| IBIS file stm32mp251_253_255_257_vfbga424.ibs
[IBIS ver] 5.1
[File name] stm32mp251_253_255_257_vfbga424.ibs
[File Rev] 1.3
[Date] 09-10-2025
[Source] Data Created at STMicroelectronics
[Notes]  File originated from ELDO simulations.
[Disclaimer]  This information is for modeling purpose only and is
   not guaranted. The information is subject to change without
   notice.
[Copyright] Copyright 2025 STMicroelectronics Inc.
|   Component stm32mp251_253_255_257_vfbga424
[Component] stm32mp25_505_tfbga14x14_424
[Manufacturer] stm32mp251_253_255_257_vfbga424
[Package]
| variable   typ   min   max
R_pkg   0.0   0.0   0.0
L_pkg   0.0H   0.0H   0.0H
C_pkg   0.0F   0.0F   0.0F
[Pin]  signal_name   model_name   R_pin   L_pin   C_pin
1A1  VSS  gnd
1A3  VSS  gnd
1A5  VSS  gnd
1A7  VSS  gnd
1A9  VSS  gnd
1A11  VSS  gnd
1B2  VSS  gnd
1B4  VSS  gnd
1B6  VSS  gnd
1B8  VSS  gnd
1B10  VSS  gnd
1B12  VSS  gnd
1C1  VDDCORE  nc
1C3  VDDCORE  nc
1C5  VDDCORE  nc
1C7  VDDCPU  nc
1C9  VDDCPU  nc
1C11  VDDQDDR  power
1D2  VDDCORE  nc
1D4  VDDCORE  nc
1D6  VDDCPU  nc
1D8  VDDCPU  nc
1D10  VDDCPU  nc
1D12  VDDQDDR  power
1E1  VDDA18PLL3  nc
1E3  VDDCORE  nc
1E5  VDDCORE  nc
1E7  VSS  gnd
1E9  VSS  gnd
1E11  VDDQDDR  power
1F2  VDDCORE  nc
1F4  VDDCORE  nc
1F6  VSS  gnd
1F8  VSS  gnd
1F10  VSS  gnd
1F12  VDDQDDR  power
1G1  VSS  gnd
1G3  VSS  gnd
1G5  VSS  gnd
1G7  VDDGPU  nc
1G9  VDDGPU  nc
1G11  VSS  gnd
1H2  VSS  gnd
1H4  VSS  gnd
1H6  VDDGPU  nc
1H8  VDDGPU  nc
1H10  VDDGPU  nc
1H12  VSS  gnd
1J1  VSS  gnd
1J3  VSS  gnd
1J5  VSS  gnd
1J7  VSS  gnd
1J9  VSS  gnd
1J11  VSS  gnd
1K2  VSS  gnd
1K4  VSS  gnd
1K6  VSS  gnd
1K8  VSS  gnd
1K10  VSS  gnd
1K12  VSS  gnd
1L1  VDD  power
1L3  VDD  power
1L5  VDD  power
1L7  VDDGPU  nc
1L9  VDDGPU  nc
1L11  VDDQDDR  power
1M2  VDD  power
1M4  VDD  power
1M6  VDDGPU  nc
1M8  VDDGPU  nc
1M10  VDDGPU  nc
1M12  VDDQDDR  power
A1  VSS  gnd
A2  VSS  gnd
A3  CSI_D0N  DPHY_IBIS_L1
A6  DSI_D3P  DPHY_IBIS
A7  DSI_D2N  DPHY_IBIS
A10  DSI_D1N  DPHY_IBIS
A11  PB11  io8_tt
A14  PB2  io8_tt
A15  PD11  io8_tt_i3c
A18  PD6  io8_tt
A19  PD1  io8_tt
A22  PE6  io8_tt
A23  PE9  io8_tt
A26  PB13  io8_tt
A27  VSS  gnd
AA1  OSC32_OUT  isudq_tt
AA2  OSC32_IN  isudq_tt
AA3  BOOT1  isudq_tt
AA5  JTCK_SWCLK  io8_tt
AA7  PG3  io8_tt
AA9  PC3  io8_tt
AA11  PF5  io8_tt
AA13  PH9  io8_tt
AA15  PF0  io8_tt_i3c
AA17  PA8  io8_tt_i3c
AA19  UCPD1_CC2  nc
AA21  DDR_A30  mal4drv20_PAD
AA23  DDR_A27  mal4drv20_PAD
AA25  DDR_DQS0P  mal4drv27_PAD
AA26  DDR_DQS0N  mal4drv27_PAD
AB1  BOOT2  isudq_tt
AB2  BOOT3  isudq_tt
AB3  VDDA18AON  power
AB4  PWR_CPUON  io8_tt
AB6  VDDA18ADC  power
AB8  PF7  io8_tt
AB10  PC6  io8_tt_i3c
AB12  PA14  io8_tt
AB14  PC0  io8_tt
AB16  PH4  io8_tt
AB18  UCPD1_CC1  nc
AB20  VDDCOMBOPHY  nc
AB22  VDDCOMBOPHYTX  nc
AB24  DDR_A26  mal4drv20_PAD
AB25  DDR_DQM0  mal4drv27_PAD
AB26  DDR_DQ0  mal4drv27_PAD
AB27  DDR_DQ2  mal4drv27_PAD
AC2  JTDO_TRACESWO  io8_tt
AC3  VSSAON  gnd
AC5  VSSA  nc
AC7  PF6  io8_tt
AC9  PC4  io8_tt
AC11  VSS  gnd
AC13  PA12  io8_tt_i3c
AC15  PF2  io8_tt_i3c
AC17  PH2  io8_tt_i3c
AC19  PA1  io8_tt_i3c
AC21  VDDPCIECLK  nc
AC23  DDR_A28  mal4drv20_PAD
AC25  DDR_A7  mal4drv20_PAD
AC26  DDR_DQ1  mal4drv27_PAD
AC27  DDR_DQ3  mal4drv27_PAD
AD3  PWR_ON  io8_tt
AD4  PG1  io8_tt_i3c
AD6  PG4  io8_tt
AD8  PC11  io8_tt
AD10  PC5  io8_tt_i3c
AD12  PA11  io8_tt
AD14  PA13  io8_tt
AD16  PH8  io8_tt
AD18  PA3  io8_tt_i3c
AD20  USB3DR_VBUS  nc
AD22  VDDA18USB  power
AD24  COMBOPHY_TX1N  synopsys_usb3_tx
AD25  DDR_A1  mal4drv20_PAD
AE1  NRST  nc
AE2  JTMS_SWDIO  io8_tt
AE3  JTDI  io8_tt
AE4  PF11  io8_tt
AE5  PF10  io8_tt
AE6  PB15  io8_tt
AE7  PC12  io8_tt_i3c
AE8  PF9  io8_tt
AE9  PC9  io8_tt
AE10  PF8  io8_tt
AE11  PF1  io8_tt
AE12  PC2  io8_tt
AE13  PA15  io8_tt_i3c
AE14  PH11  io8_tt
AE15  PA10  io8_tt
AE16  PH7  io8_tt_i3c
AE17  PA5  io8_tt
AE18  PA7  io8_tt
AE19  PH3  io8_tt_i3c
AE20  USBH_HS_TXRTUNE  nc
AE21  VDD33USB  power
AE22  VDD33UCPD  nc
AE23  VDDA18COMBOPHY  power
AE24  COMBOPHY_TX1P  synopsys_usb3_tx
AE25  PCIE_CLKINP  nc
AE26  PCIE_CLKINN  nc
AF1  PWR_LP  io8_tt
AF2  OSC_OUT  isudq_tt
AF3  NJTRST  io8_tt
AF5  PA0  io8_tt
AF6  VREFN  nc
AF7  PG0  io8_tt_i3c
AF9  PC7  io8_tt
AF10  PF4  io8_tt
AF11  PF3  io8_tt
AF13  PH12  io8_tt
AF14  PH10  io8_tt
AF15  PA9  io8_tt
AF17  PA2  io8_tt_i3c
AF18  PA6  io8_tt
AF19  PH6  io8_tt_i3c
AF21  USBH_HS_DP  USB2_HS_IBIS
AF22  USB3DR_DP  USB2_HS_IBIS
AF23  USB3DR_TXRTUNE  nc
AF25  COMBOPHY_RX1N  synopsys_usb3_rx
AF26  PCIE_CLKOUTP  nc
AF27  COMBOPHY_REXT  nc
AG1  VSS  gnd
AG2  OSC_IN  isudq_tt
AG5  PG2  io8_tt_i3c
AG6  VREFP  nc
AG9  PC8  io8_tt
AG10  PC10  io8_tt
AG13  PH13  io8_tt
AG14  PC1  io8_tt_i3c
AG17  PA4  io8_tt
AG18  PH5  io8_tt
AG21  USBH_HS_DM  USB2_HS_IBIS
AG22  USB3DR_DM  USB2_HS_IBIS
AG25  COMBOPHY_RX1P  synopsys_usb3_rx
AG26  PCIE_CLKOUTN  nc
AG27  VSS  gnd
B1  LVDS2_D0P  nc
B2  LVDS2_D0N  nc
B3  CSI_D0P  DPHY_IBIS_L1
B5  CSI_D1P  DPHY_IBIS_L1
B6  DSI_D3N  DPHY_IBIS
B7  DSI_D2P  DPHY_IBIS
B9  DSI_D0P  DPHY_IBIS
B10  DSI_D1P  DPHY_IBIS
B11  PB10  io8_tt
B13  PB0  io8_tt
B14  PB3  io8_tt
B15  PB4  io8_tt_i3c
B17  PD0  io8_tt
B18  PD5  io8_tt
B19  PE0  io8_tt
B21  PE4  io8_tt
B22  PE7  io8_tt
B23  PE11  io8_tt
B25  PE14  io8_tt
B26  PD12  io8_tt
B27  PI11  io8_tt
C2  LVDS2_D1P  nc
C3  LVDS2_D1N  nc
C4  CSI_CKP  DPHY_IBIS_L1
C5  CSI_D1N  DPHY_IBIS_L1
C6  VSS  gnd
C7  DSI_CKP  DPHY_IBIS
C8  DSI_CKN  DPHY_IBIS
C9  DSI_D0N  DPHY_IBIS
C10  VSS  gnd
C11  PB7  io8_tt
C12  PB1  io8_tt
C13  PB6  io8_tt
C14  PB5  io8_tt_i3c
C15  PD9  io8_tt
C16  PD8  io8_tt
C17  PD10  io8_tt_i3c
C18  PD4  io8_tt
C19  PE1  io8_tt
C20  PE2  io8_tt
C21  PE3  io8_tt
C22  PE5  io8_tt
C23  PE8  io8_tt
C24  PE13  io8_tt
C25  PE12  io8_tt
C26  PB12  io8_tt
C27  PB14  io8_tt
D3  LVDS2_D2N  nc
D4  CSI_CKN  DPHY_IBIS_L1
D6  DSI_REXT  nc
D8  PB8  io8_tt
D10  VDDIO3  power
D12  PD2  io8_tt
D14  VDDIO1  power
D16  PI10  io8_tt
D18  VDDIO2  power
D20  PD7  io8_tt
D22  PE10  io8_tt
D24  PE15  io8_tt
D25  PD13  io8_tt
E1  LVDS2_D3P  nc
E2  LVDS2_D3N  nc
E3  LVDS2_D2P  nc
E5  VDDCSI  nc
E7  VSS  gnd
E9  VDDIO4  power
E11  VDDIO3  power
E13  VDDIO1  power
E15  PD15  io8_tt_i3c
E17  VDDIO2  power
E19  PD14  io8_tt_i3c
E21  DDR_RESETN  nc
E23  DDR_A23  mal4drv20_PAD
E25  DDR_DQ19  mal4drv27_PAD
E26  DDR_DQ17  mal4drv27_PAD
F1  LVDS2_D4P  nc
F2  LVDS2_D4N  nc
F3  VSS  gnd
F4  VDDLVDS  nc
F6  CSI_REXT  nc
F8  VDDDSI  nc
F10  PB9  io8_tt
F12  VSS  gnd
F14  VSS  gnd
F16  VSS  gnd
F18  VDDCPU  nc
F20  VDDA18DDR  nc
F22  DDR_A22  mal4drv20_PAD
F24  DDR_DQ18  mal4drv27_PAD
F25  DDR_DQ16  mal4drv27_PAD
F26  DDR_DQS2N  mal4drv27_PAD
F27  DDR_DQS2P  mal4drv27_PAD
G2  LVDS1_D0P  nc
G3  LVDS1_D0N  nc
G5  VDDA18LVDS  power
G7  VDDA18CSI  power
G9  VDDA18DSI  power
G11  VDDIO4  power
G13  PD3  io8_tt
G15  VDDCPU  nc
G17  VDDCPU  nc
G19  VDDA18PLL1  nc
G21  DDR_VREF  nc
G23  DDR_A18  mal4drv20_PAD
G25  DDR_DQ23  mal4drv27_PAD
G26  DDR_DQ22  mal4drv27_PAD
G27  DDR_DQM2  mal4drv27_PAD
H3  LVDS1_D1P  nc
H4  LVDS1_D1N  nc
H6  VDDA18PLL2  nc
H22  DDR_A21  mal4drv20_PAD
H24  DDR_A17  mal4drv20_PAD
H25  DDR_DQ21  mal4drv27_PAD
J1  LVDS1_D2P  nc
J2  LVDS1_D2N  nc
J3  PI6  io8_tt
J5  PI7  io8_tt
J7  VSS  gnd
J21  DDR_A20  mal4drv20_PAD
J23  DDR_A16  mal4drv20_PAD
J25  DDR_DQ20  mal4drv27_PAD
J26  DDR_DQ24  mal4drv27_PAD
K1  LVDS1_D4P  nc
K2  LVDS1_D4N  nc
K3  VSS  gnd
K4  PI5  io8_tt
K6  PG15  io8_tt
K22  DDR_ZQ  nc
K24  DDR_A13  mal4drv20_PAD
K25  DDR_DQ25  mal4drv27_PAD
K26  DDR_DQ26  mal4drv27_PAD
K27  DDR_DQ27  mal4drv27_PAD
L2  LVDS1_D3P  nc
L3  LVDS1_D3N  nc
L5  PG8  io8_tt
L7  PI0  io8_tt
L21  DDR_A19  mal4drv20_PAD
L23  DDR_A12  mal4drv20_PAD
L25  DDR_DQ28  mal4drv27_PAD
L26  DDR_DQS3P  mal4drv27_PAD
L27  DDR_DQS3N  mal4drv27_PAD
M3  PG9  io8_tt
M4  PG10  io8_tt
M6  PI1  io8_tt_i3c
M22  VDDQDDR  power
M24  DDR_A14  mal4drv20_PAD
M25  DDR_DQM3  mal4drv27_PAD
N1  PG14  io8_tt
N2  PG11  io8_tt
N3  PG12  io8_tt
N5  PI2  io8_tt
N7  PI3  io8_tt
N21  VDDQDDR  power
N23  DDR_A15  mal4drv20_PAD
N25  DDR_DQ29  mal4drv27_PAD
N26  DDR_DQ30  mal4drv27_PAD
P1  PG13  io8_tt_i3c
P2  PF13  io8_tt
P3  PF14  io8_tt
P4  PF12  io8_tt
P6  PI4  io8_tt
P22  DDR_A3  mal4drv20_PAD
P24  DDR_A11  mal4drv20_PAD
P25  DDR_DQ31  mal4drv27_PAD
P26  DDR_DQ11  mal4drv27_PAD
P27  DDR_DQ10  mal4drv27_PAD
R2  PF15  io8_tt
R3  PG5  io8_tt_i3c
R5  PZ5  io8_tt
R7  V08CAP  nc
R21  VDDQDDR  power
R23  DDR_A10  mal4drv20_PAD
R25  DDR_DQS1N  mal4drv27_PAD
R26  DDR_DQ9  mal4drv27_PAD
R27  DDR_DQ8  mal4drv27_PAD
T3  PG6  io8_tt_i3c
T4  PZ0  io8_tt_i3c
T6  VBAT  power
T22  DDR_A9  mal4drv20_PAD
T24  DDR_A5  mal4drv20_PAD
T25  DDR_DQS1P  mal4drv27_PAD
U1  PI9  io8_tt
U2  PG7  io8_tt
U3  PZ9  io8_tt_i3c
U5  PI8  io8_tt
U7  PZ1  io8_tt_i3c
U21  DDR_A0  mal4drv20_PAD
U23  DDR_A4  mal4drv20_PAD
U25  DDR_DQ15  mal4drv27_PAD
U26  DDR_DQM1  mal4drv27_PAD
V1  PZ8  io8_tt
V2  PZ7  io8_tt
V3  PZ4  io8_tt_i3c
V4  PZ6  io8_tt
V6  VSS  gnd
V22  DDR_A8  mal4drv20_PAD
V24  DDR_A2  mal4drv20_PAD
V25  DDR_DQ14  mal4drv27_PAD
V26  DDR_DQ12  mal4drv27_PAD
V27  DDR_DQ13  mal4drv27_PAD
W2  PDR_ON  nc
W3  NRSTC1MS  io8_tt
W5  PZ2  io8_tt_i3c
W7  PC13  io8_tt
W21  DDR_A25  mal4drv20_PAD
W23  DDR_A31  mal4drv20_PAD
W25  DDR_DQ4  mal4drv27_PAD
W26  DDR_DQ6  mal4drv27_PAD
W27  DDR_DQ5  mal4drv27_PAD
Y3  BOOT0  isudq_tt
Y4  VSS  gnd
Y6  PZ3  io8_tt_i3c
Y22  DDR_A29  mal4drv20_PAD
Y24  DDR_A6  mal4drv20_PAD
Y25  DDR_DQ7  mal4drv27_PAD
[Package Model]   505-fcbga-14x14-424-240118v2
[Pin Mapping]   pulldown_ref   pullup_ref   | Comment
1A1  gnd  nc
1A3  gnd  nc
1A5  gnd  nc
1A7  gnd  nc
1A9  gnd  nc
1A11  gnd  nc
1B2  gnd  nc
1B4  gnd  nc
1B6  gnd  nc
1B8  gnd  nc
1B10  gnd  nc
1B12  gnd  nc
1C1  nc  nc
1C3  nc  nc
1C5  nc  nc
1C7  nc  nc
1C9  nc  nc
1C11  nc  vddqddr
1D2  nc  nc
1D4  nc  nc
1D6  nc  nc
1D8  nc  nc
1D10  nc  nc
1D12  nc  vddqddr
1E1  nc  nc
1E3  nc  nc
1E5  nc  nc
1E7  gnd  nc
1E9  gnd  nc
1E11  nc  vddqddr
1F2  nc  nc
1F4  nc  nc
1F6  gnd  nc
1F8  gnd  nc
1F10  gnd  nc
1F12  nc  vddqddr
1G1  gnd  nc
1G3  gnd  nc
1G5  gnd  nc
1G7  nc  nc
1G9  nc  nc
1G11  gnd  nc
1H2  gnd  nc
1H4  gnd  nc
1H6  nc  nc
1H8  nc  nc
1H10  nc  nc
1H12  gnd  nc
1J1  gnd  nc
1J3  gnd  nc
1J5  gnd  nc
1J7  gnd  nc
1J9  gnd  nc
1J11  gnd  nc
1K2  gnd  nc
1K4  gnd  nc
1K6  gnd  nc
1K8  gnd  nc
1K10  gnd  nc
1K12  gnd  nc
1L1  nc  vdd
1L3  nc  vdd
1L5  nc  vdd
1L7  nc  nc
1L9  nc  nc
1L11  nc  vddqddr
1M2  nc  vdd
1M4  nc  vdd
1M6  nc  nc
1M8  nc  nc
1M10  nc  nc
1M12  nc  vddqddr
A1  gnd  nc
A2  gnd  nc
A3  gnd  VDDA18CSI
A6  gnd  VDDA18DSI
A7  gnd  VDDA18DSI
A10  gnd  VDDA18DSI
A11  gnd  vddio4
A14  gnd  vddio4
A15  gnd  vddio3
A18  gnd  vddio3
A19  gnd  vddio3
A22  gnd  vddio2
A23  gnd  vddio2
A26  gnd  vdd
A27  gnd  nc
AA1  gnd  vdd  | Depending on IO usage
| AA1  gnd  vsw  | Depending on IO usage
AA2  gnd  vdd  | Depending on IO usage
| AA2  gnd  vsw  | Depending on IO usage
AA3  gnd  vdd
AA5  gnd  vdd
AA7  gnd  vdd  | Depending on IO usage
| AA7  gnd  vsw  | Depending on IO usage
AA9  gnd  vdd  | Depending on IO usage
| AA9  gnd  vsw  | Depending on IO usage
AA11  gnd  vdd
AA13  gnd  vdd
AA15  gnd  vdd
AA17  gnd  vdd
AA19  nc  nc
AA21  gnd  vddqddr
AA23  gnd  vddqddr
AA25  gnd  vddqddr
AA26  gnd  vddqddr
AB1  gnd  vdd
AB2  gnd  vdd
AB3  nc  vdda18aon
AB4  gnd  vdd
AB6  nc  vdda18adc
AB8  gnd  vdd  | Depending on IO usage
| AB8  gnd  vsw  | Depending on IO usage
AB10  gnd  vdd
AB12  gnd  vdd
AB14  gnd  vdd
AB16  gnd  vdd
AB18  nc  nc
AB20  nc  nc
AB22  nc  nc
AB24  gnd  vddqddr
AB25  gnd  vddqddr
AB26  gnd  vddqddr
AB27  gnd  vddqddr
AC2  gnd  vdd
AC3  gnd_aon  nc
AC5  nc  nc
AC7  gnd  vdd  | Depending on IO usage
| AC7  gnd  vsw  | Depending on IO usage
AC9  gnd  vdd  | Depending on IO usage
| AC9  gnd  vsw  | Depending on IO usage
AC11  gnd  nc
AC13  gnd  vdd
AC15  gnd  vdd
AC17  gnd  vdd
AC19  gnd  vdd
AC21  nc  nc
AC23  gnd  vddqddr
AC25  gnd  vddqddr
AC26  gnd  vddqddr
AC27  gnd  vddqddr
AD3  gnd  vdd
AD4  gnd  vdd  | Depending on IO usage
| AD4  gnd  vsw  | Depending on IO usage
AD6  gnd  vdd
AD8  gnd  vdd
AD10  gnd  vdd  | Depending on IO usage
| AD10  gnd  vsw  | Depending on IO usage
AD12  gnd  vdd
AD14  gnd  vdd
AD16  gnd  vdd
AD18  gnd  vdd
AD20  nc  nc
AD22  nc  vdda18usb
AD24  gnd  vdda18combophy
AD25  gnd  vddqddr
AE1  nc  nc
AE2  gnd  vdd
AE3  gnd  vdd
AE4  gnd  vdd
AE5  gnd  vdd
AE6  gnd  vdd
AE7  gnd  vdd
AE8  gnd  vdd
AE9  gnd  vdd
AE10  gnd  vdd
AE11  gnd  vdd
AE12  gnd  vdd
AE13  gnd  vdd
AE14  gnd  vdd
AE15  gnd  vdd
AE16  gnd  vdd
AE17  gnd  vdd
AE18  gnd  vdd
AE19  gnd  vdd
AE20  nc  nc
AE21  nc  VDD33USB
AE22  nc  nc
AE23  nc  vdda18combophy
AE24  gnd  vdda18combophy
AE25  nc  nc
AE26  nc  nc
AF1  gnd  vdd
AF2  gnd_aon  vdda18aon
AF3  gnd  vdd
AF5  gnd  vdd
AF6  nc  nc
AF7  gnd  vdd
AF9  gnd  vdd
AF10  gnd  vdd
AF11  gnd  vdd
AF13  gnd  vdd
AF14  gnd  vdd
AF15  gnd  vdd
AF17  gnd  vdd
AF18  gnd  vdd
AF19  gnd  vdd
AF21  gnd  VDD33USB
AF22  gnd  VDD33USB
AF23  nc  nc
AF25  gnd  vdda18combophy
AF26  nc  nc
AF27  nc  nc
AG1  gnd  nc
AG2  gnd_aon  vdda18aon
AG5  gnd  vdd
AG6  nc  nc
AG9  gnd  vdd
AG10  gnd  vdd
AG13  gnd  vdd
AG14  gnd  vdd
AG17  gnd  vdd
AG18  gnd  vdd
AG21  gnd  VDD33USB
AG22  gnd  VDD33USB
AG25  gnd  vdda18combophy
AG26  nc  nc
AG27  gnd  nc
B1  nc  nc
B2  nc  nc
B3  gnd  VDDA18CSI
B5  gnd  VDDA18CSI
B6  gnd  VDDA18DSI
B7  gnd  VDDA18DSI
B9  gnd  VDDA18DSI
B10  gnd  VDDA18DSI
B11  gnd  vddio4
B13  gnd  vddio4
B14  gnd  vddio4
B15  gnd  vddio4
B17  gnd  vddio3
B18  gnd  vddio3
B19  gnd  vddio1
B21  gnd  vddio1
B22  gnd  vddio2
B23  gnd  vddio2
B25  gnd  vddio2
B26  gnd  vdd
B27  gnd  vdd
C2  nc  nc
C3  nc  nc
C4  gnd  VDDA18CSI
C5  gnd  VDDA18CSI
C6  gnd  nc
C7  gnd  VDDA18DSI
C8  gnd  VDDA18DSI
C9  gnd  VDDA18DSI
C10  gnd  nc
C11  gnd  vddio4
C12  gnd  vddio4
C13  gnd  vddio4
C14  gnd  vddio4
C15  gnd  vddio3
C16  gnd  vddio3
C17  gnd  vddio3
C18  gnd  vddio3
C19  gnd  vddio1
C20  gnd  vddio1
C21  gnd  vddio1
C22  gnd  vddio1
C23  gnd  vddio2
C24  gnd  vddio2
C25  gnd  vddio2
C26  gnd  vdd
C27  gnd  vdd
D3  nc  nc
D4  gnd  VDDA18CSI
D6  nc  nc
D8  gnd  vddio4
D10  nc  vddio3
D12  gnd  vddio3
D14  nc  vddio1
D16  gnd  vdd
D18  nc  vddio2
D20  gnd  vddio3
D22  gnd  vddio2
D24  gnd  vddio2
D25  gnd  vdd
E1  nc  nc
E2  nc  nc
E3  nc  nc
E5  nc  nc
E7  gnd  nc
E9  nc  vddio4
E11  nc  vddio3
E13  nc  vddio1
E15  gnd  vdd
E17  nc  vddio2
E19  gnd  vdd
E21  nc  nc
E23  gnd  vddqddr
E25  gnd  vddqddr
E26  gnd  vddqddr
F1  nc  nc
F2  nc  nc
F3  gnd  nc
F4  nc  nc
F6  nc  nc
F8  nc  nc
F10  gnd  vddio4
F12  gnd  nc
F14  gnd  nc
F16  gnd  nc
F18  nc  nc
F20  nc  nc
F22  gnd  vddqddr
F24  gnd  vddqddr
F25  gnd  vddqddr
F26  gnd  vddqddr
F27  gnd  vddqddr
G2  nc  nc
G3  nc  nc
G5  nc  vdda18lvds
G7  nc  VDDA18CSI
G9  nc  VDDA18DSI
G11  nc  vddio4
G13  gnd  vddio3
G15  nc  nc
G17  nc  nc
G19  nc  nc
G21  nc  nc
G23  gnd  vddqddr
G25  gnd  vddqddr
G26  gnd  vddqddr
G27  gnd  vddqddr
H3  nc  nc
H4  nc  nc
H6  nc  nc
H22  gnd  vddqddr
H24  gnd  vddqddr
H25  gnd  vddqddr
J1  nc  nc
J2  nc  nc
J3  gnd  vdd
J5  gnd  vdd
J7  gnd  nc
J21  gnd  vddqddr
J23  gnd  vddqddr
J25  gnd  vddqddr
J26  gnd  vddqddr
K1  nc  nc
K2  nc  nc
K3  gnd  nc
K4  gnd  vdd
K6  gnd  vdd
K22  nc  nc
K24  gnd  vddqddr
K25  gnd  vddqddr
K26  gnd  vddqddr
K27  gnd  vddqddr
L2  nc  nc
L3  nc  nc
L5  gnd  vdd
L7  gnd  vdd
L21  gnd  vddqddr
L23  gnd  vddqddr
L25  gnd  vddqddr
L26  gnd  vddqddr
L27  gnd  vddqddr
M3  gnd  vdd
M4  gnd  vdd
M6  gnd  vdd
M22  nc  vddqddr
M24  gnd  vddqddr
M25  gnd  vddqddr
N1  gnd  vdd
N2  gnd  vdd
N3  gnd  vdd
N5  gnd  vdd
N7  gnd  vdd
N21  nc  vddqddr
N23  gnd  vddqddr
N25  gnd  vddqddr
N26  gnd  vddqddr
P1  gnd  vdd
P2  gnd  vdd
P3  gnd  vdd
P4  gnd  vdd
P6  gnd  vdd
P22  gnd  vddqddr
P24  gnd  vddqddr
P25  gnd  vddqddr
P26  gnd  vddqddr
P27  gnd  vddqddr
R2  gnd  vdd
R3  gnd  vdd
R5  gnd  vdd  | Depending on IO usage
| R5  gnd  vsw  | Depending on IO usage
R7  nc  nc
R21  nc  vddqddr
R23  gnd  vddqddr
R25  gnd  vddqddr
R26  gnd  vddqddr
R27  gnd  vddqddr
T3  gnd  vdd
T4  gnd  vdd  | Depending on IO usage
| T4  gnd  vsw  | Depending on IO usage
T6  nc  vsw
T22  gnd  vddqddr
T24  gnd  vddqddr
T25  gnd  vddqddr
U1  gnd  vdd
U2  gnd  vdd
U3  gnd  vdd
U5  gnd  vdd  | Depending on IO usage
| U5  gnd  vsw  | Depending on IO usage
U7  gnd  vdd  | Depending on IO usage
| U7  gnd  vsw  | Depending on IO usage
U21  gnd  vddqddr
U23  gnd  vddqddr
U25  gnd  vddqddr
U26  gnd  vddqddr
V1  gnd  vdd
V2  gnd  vdd
V3  gnd  vdd  | Depending on IO usage
| V3  gnd  vsw  | Depending on IO usage
V4  gnd  vdd  | Depending on IO usage
| V4  gnd  vsw  | Depending on IO usage
V6  gnd  nc
V22  gnd  vddqddr
V24  gnd  vddqddr
V25  gnd  vddqddr
V26  gnd  vddqddr
V27  gnd  vddqddr
W2  nc  nc
W3  gnd  vdd
W5  gnd  vdd  | Depending on IO usage
| W5  gnd  vsw  | Depending on IO usage
W7  gnd  vdd  | Depending on IO usage
| W7  gnd  vsw  | Depending on IO usage
W21  gnd  vddqddr
W23  gnd  vddqddr
W25  gnd  vddqddr
W26  gnd  vddqddr
W27  gnd  vddqddr
Y3  gnd  vdd
Y4  gnd  nc
Y6  gnd  vdd  | Depending on IO usage
| Y6  gnd  vsw  | Depending on IO usage
Y22  gnd  vddqddr
Y24  gnd  vddqddr
Y25  gnd  vddqddr
[Diff Pin]   inv_pin   vdiff   tdelay_typ   tdelay_min   tdelay_max
U23   T24   0.320V   0ns   NA   NA   |CKA
|J23   H24   0.320V   0ns   NA   NA   |CKB only in LPDDR4 32 bit
AA25   AA26   0.320V   0ns   NA   NA   |DQS0
T25   R25   0.320V   0ns   NA   NA   |DQS1
F27   F26   0.320V   0ns   NA   NA   |DQS2
L26   L27   0.320V   0ns   NA   NA   |DQS3
AG25   AF25   NA   NA   NA   NA
AE24   AD24   NA   NA   NA   NA
C4   D4   NA   NA   NA   NA
B3   A3   NA   NA   NA   NA
B5   C5   NA   NA   NA   NA
C7   C8   NA   NA   NA   NA  |DSI CKP CKN
B9   C9   400.000mV   0ns   NA   NA   |D0P D0N
B10   A10   400.000mV   0ns   NA   NA   |D1P D1N
B7   A7   400.000mV   0ns   NA   NA   |D2P D2N
A6   B6   400.000mV   0ns   NA   NA   |D3P D3N
G2   G3   NA   NA   NA   NA
H3   H4   NA   NA   NA   NA
J1   J2   NA   NA   NA   NA
L2   L3   NA   NA   NA   NA
K1   K2   NA   NA   NA   NA
B1   B2   NA   NA   NA   NA
C2   C3   NA   NA   NA   NA
E3   D3   NA   NA   NA   NA
E1   E2   NA   NA   NA   NA
F1   F2   NA   NA   NA   NA
AE25   AE26   NA   NA   NA   NA
AF26   AG26   NA   NA   NA   NA
AF22   AG22   NA   NA   NA   NA   |USB3DR_DP _DM
AF21   AG21   NA   NA   NA   NA   |USBH_HS_DP _DM
[Model Selector] DPHY_IBIS_L1
DPHY_RX_2P5G_L1   DPHY HSRX model at 2.5Gbps for lane 1
DPHY_RX_1P5G_L1   DPHY HSRX model at 1.5Gbps for lane 1
[Model Selector] DPHY_IBIS
DPHY_TX_2P5G   DPHY HSTX model at 2.5Gbps
DPHY_TX_1P5G   DPHY HSTX model at 1.5Gbps
[Model Selector] USB2_HS_IBIS
USB2_HSRX   USB2 HSRX model
USB2_HSTX_00_0_01_0011_11   TuningBits_AMP_PULSE_RISE_REF_XV=00_0_01_0011_11
USB2_HSTX_00_0_10_0101_11   TuningBits_AMP_PULSE_RISE_REF_XV=00_0_10_0101_11
USB2_HSTX_00_0_11_0111_11   TuningBits_AMP_PULSE_RISE_REF_XV=00_0_11_0111_11
USB2_HSTX_00_1_01_0011_11   TuningBits_AMP_PULSE_RISE_REF_XV=00_1_01_0011_11
USB2_HSTX_00_1_10_0101_11   TuningBits_AMP_PULSE_RISE_REF_XV=00_1_10_0101_11
USB2_HSTX_00_1_11_0111_11   TuningBits_AMP_PULSE_RISE_REF_XV=00_1_11_0111_11
USB2_HSTX_01_0_01_0011_11   TuningBits_AMP_PULSE_RISE_REF_XV=01_0_01_0011_11
USB2_HSTX_01_0_10_0101_11   TuningBits_AMP_PULSE_RISE_REF_XV=01_0_10_0101_11
USB2_HSTX_01_0_11_0111_11   TuningBits_AMP_PULSE_RISE_REF_XV=01_0_11_0111_11
USB2_HSTX_01_1_01_0011_11   TuningBits_AMP_PULSE_RISE_REF_XV=01_1_01_0011_11
USB2_HSTX_01_1_10_0101_11   TuningBits_AMP_PULSE_RISE_REF_XV=01_1_10_0101_11
USB2_HSTX_01_1_11_0111_11   TuningBits_AMP_PULSE_RISE_REF_XV=01_1_11_0111_11
USB2_HSTX_10_0_01_0011_11   TuningBits_AMP_PULSE_RISE_REF_XV=10_0_01_0011_11
USB2_HSTX_10_0_10_0101_11   TuningBits_AMP_PULSE_RISE_REF_XV=10_0_10_0101_11
USB2_HSTX_10_0_11_0111_11   TuningBits_AMP_PULSE_RISE_REF_XV=10_0_11_0111_11
USB2_HSTX_10_1_01_0011_11   TuningBits_AMP_PULSE_RISE_REF_XV=10_1_01_0011_11
USB2_HSTX_10_1_10_0101_11   TuningBits_AMP_PULSE_RISE_REF_XV=10_1_10_0101_11
USB2_HSTX_10_1_11_0111_11   TuningBits_AMP_PULSE_RISE_REF_XV=10_1_11_0111_11
[Model Selector] io8_tt
io8_tt_ls_3v3   "GPIO - 3V tolerant - 3.3V range - Low speed"
io8_tt_ms_3v3   "GPIO - 3V tolerant - 3.3V range - Med speed"
io8_tt_fs_3v3   "GPIO - 3V tolerant - 3.3V range - Fast speed"
io8_tt_hs_3v3   "GPIO - 3V tolerant - 3.3V range - High speed"
io8_tt_hslv_ls_1v8   "GPIO HSLV - 3V tolerant - 1.8V range - Low speed"
io8_tt_hslv_ms_1v8   "GPIO HSLV - 3V tolerant - 1.8V range - Med speed"
io8_tt_hslv_fs_1v8   "GPIO HSLV - 3V tolerant - 1.8V range - Fast speed"
io8_tt_hslv_hs_1v8   "GPIO HSLV - 3V tolerant - 1.8V range - High speed"
[Model Selector] io8_tt_i3c
io8_tt_ls_3v3   "GPIO - 3V tolerant - 3.3V range - Low speed"
io8_tt_ms_3v3   "GPIO - 3V tolerant - 3.3V range - Med speed"
io8_tt_fs_3v3   "GPIO - 3V tolerant - 3.3V range - Fast speed"
io8_tt_hs_3v3   "GPIO - 3V tolerant - 3.3V range - High speed"
io8_tt_hslv_ls_1v8   "GPIO HSLV - 3V tolerant - 1.8V range - Low speed"
io8_tt_hslv_ms_1v8   "GPIO HSLV - 3V tolerant - 1.8V range - Med speed"
io8_tt_hslv_fs_1v8   "GPIO HSLV - 3V tolerant - 1.8V range - Fast speed"
io8_tt_hslv_hs_1v8   "GPIO HSLV - 3V tolerant - 1.8V range - High speed"
io8_tt_i3c_3v3   "GPIO - 3V tolerant - 3.3V range - Open drain"
[Model Selector] isudq_tt
isudq_tt_1v8   "Input Buffer - 3V tolerant - 1.8V range"
isudq_tt_3v3   "Input Buffer - 3V tolerant - 3.3V range"
[Model Selector]   mal4drv20_PAD
mal4drv20_d3l_40   DDR3L mal4drv20 cell  Z0=40-Ohm Driver
mal4drv20_d3l_60   DDR3L mal4drv20 cell  Z0=60-Ohm Driver
mal4drv20_d3l_120   DDR3L mal4drv20 cell  Z0=120-Ohm Driver
mal4drv20_d3_20   DDR3 mal4drv20 cell  Z0=20-Ohm Driver
mal4drv20_d3_24   DDR3 mal4drv20 cell  Z0=24-Ohm Driver
mal4drv20_d3_30   DDR3 mal4drv20 cell  Z0=30-Ohm Driver
mal4drv20_d3_40   DDR3 mal4drv20 cell  Z0=40-Ohm Driver
mal4drv20_d3_60   DDR3 mal4drv20 cell  Z0=60-Ohm Driver
mal4drv20_d4_20   DDR4 mal4drv20 cell  Z0=20-Ohm Driver
mal4drv20_d4_24   DDR4 mal4drv20 cell  Z0=24-Ohm Driver
mal4drv20_d4_30   DDR4 mal4drv20 cell  Z0=30-Ohm Driver
mal4drv20_d4_40   DDR4 mal4drv20 cell  Z0=40-Ohm Driver
mal4drv20_d4_60   DDR4 mal4drv20 cell  Z0=60-Ohm Driver
mal4drv20_dl4_20   LPDDR4 mal4drv20 cell  Z0=20-Ohm Driver
mal4drv20_dl4_24   LPDDR4 mal4drv20 cell  Z0=24-Ohm Driver
mal4drv20_dl4_30   LPDDR4 mal4drv20 cell  Z0=30-Ohm Driver
mal4drv20_dl4_40   LPDDR4 mal4drv20 cell  Z0=40-Ohm Driver
mal4drv20_dl4_60   LPDDR4 mal4drv20 cell  Z0=60-Ohm Driver
[Model Selector]   mal4drv27_PAD
mal4drv27_d3l_40   DDR3L mal4drv27 cell  Z0=40-Ohm Driver
mal4drv27_d3l_48   DDR3L mal4drv27 cell  Z0=48-Ohm Driver
mal4drv27_d3l_60   DDR3L mal4drv27 cell  Z0=60-Ohm Driver
mal4drv27_d3l_80   DDR3L mal4drv27 cell  Z0=80-Ohm Driver
mal4drv27_d3l_120   DDR3L mal4drv27 cell  Z0=120-Ohm Driver
mal4drv27_d3l_240   DDR3L mal4drv27 cell  Z0=240-Ohm Driver
mal4drv27_d3l_odt120   DDR3L mal4drv27 cell 120-Ohm ODT Receiver
mal4drv27_d3l_odt60   DDR3L mal4drv27 cell 60-Ohm ODT Receiver
mal4drv27_d3l_odtoff   DDR3L mal4drv27 cell ODT OFF Receiver
mal4drv27_d3_28   DDR3 mal4drv27 cell  Z0=28-Ohm Driver
mal4drv27_d3_34   DDR3 mal4drv27 cell  Z0=34-Ohm Driver
mal4drv27_d3_40   DDR3 mal4drv27 cell  Z0=40-Ohm Driver
mal4drv27_d3_53   DDR3 mal4drv27 cell  Z0=53-Ohm Driver
mal4drv27_d3_odt120   DDR3 mal4drv27 cell 120-Ohm ODT Receiver
mal4drv27_d3_odt60   DDR3 mal4drv27 cell 60-Ohm ODT Receiver
mal4drv27_d4_28   DDR4 mal4drv27 cell  Z0=28-Ohm Driver
mal4drv27_d4_34   DDR4 mal4drv27 cell  Z0=34-Ohm Driver
mal4drv27_d4_40   DDR4 mal4drv27 cell  Z0=40-Ohm Driver
mal4drv27_d4_53   DDR4 mal4drv27 cell  Z0=53-Ohm Driver
mal4drv27_d4_odt120   DDR4 mal4drv27 cell 120-Ohm ODT Receiver
mal4drv27_d4_odt240   DDR4 mal4drv27 cell 240-Ohm ODT Receiver
mal4drv27_d4_odt48   DDR4 mal4drv27 cell 48-Ohm ODT Receiver
mal4drv27_d4_odt60   DDR4 mal4drv27 cell 60-Ohm ODT Receiver
mal4drv27_d4_odt80   DDR4 mal4drv27 cell 80-Ohm ODT Receiver
mal4drv27_dl4_28   LPDDR4 mal4drv27 cell  Z0=28-Ohm Driver
mal4drv27_dl4_34   LPDDR4 mal4drv27 cell  Z0=34-Ohm Driver
mal4drv27_dl4_40   LPDDR4 mal4drv27 cell  Z0=40-Ohm Driver
mal4drv27_dl4_53   LPDDR4 mal4drv27 cell  Z0=53-Ohm Driver
mal4drv27_dl4_odt48   LPDDR4 mal4drv27 cell 48-Ohm ODT Receiver
mal4drv27_dl4_odt60   LPDDR4 mal4drv27 cell 60-Ohm ODT Receiver
[Define Package Model]  505-fcbga-14x14-424-240118v2
[Manufacturer]  unknown
[OEM]  unknown
[Description]  unknown
[Number Of Pins]  332
[Pin Numbers]
| Pin Name Terminal   Net Name   Starting Node   Ending Node
Y3 | BOOT0
AA3 | BOOT1
AB1 | BOOT2
AB2 | BOOT3
AF27 | COMBOPHY_REXT
AF25 | COMBOPHY_RX1N
AG25 | COMBOPHY_RX1P
AD24 | COMBOPHY_TX1N
AE24 | COMBOPHY_TX1P
D4 | CSI_CKN
C4 | CSI_CKP
A3 | CSI_D0N
B3 | CSI_D0P
C5 | CSI_D1N
B5 | CSI_D1P
F6 | CSI_REXT
U21 | DDR_A0
AD25 | DDR_A1
V24 | DDR_A2
P22 | DDR_A3
U23 | DDR_A4
T24 | DDR_A5
Y24 | DDR_A6
AC25 | DDR_A7
V22 | DDR_A8
T22 | DDR_A9
R23 | DDR_A10
P24 | DDR_A11
L23 | DDR_A12
K24 | DDR_A13
M24 | DDR_A14
N23 | DDR_A15
J23 | DDR_A16
H24 | DDR_A17
G23 | DDR_A18
L21 | DDR_A19
J21 | DDR_A20
H22 | DDR_A21
F22 | DDR_A22
E23 | DDR_A23
W21 | DDR_A25
AB24 | DDR_A26
AA23 | DDR_A27
AC23 | DDR_A28
Y22 | DDR_A29
AA21 | DDR_A30
W23 | DDR_A31
AB26 | DDR_DQ0
AC26 | DDR_DQ1
AB27 | DDR_DQ2
AC27 | DDR_DQ3
W25 | DDR_DQ4
W27 | DDR_DQ5
W26 | DDR_DQ6
Y25 | DDR_DQ7
R27 | DDR_DQ8
R26 | DDR_DQ9
P27 | DDR_DQ10
P26 | DDR_DQ11
V26 | DDR_DQ12
V27 | DDR_DQ13
V25 | DDR_DQ14
U25 | DDR_DQ15
F25 | DDR_DQ16
E26 | DDR_DQ17
F24 | DDR_DQ18
E25 | DDR_DQ19
J25 | DDR_DQ20
H25 | DDR_DQ21
G26 | DDR_DQ22
G25 | DDR_DQ23
J26 | DDR_DQ24
K25 | DDR_DQ25
K26 | DDR_DQ26
K27 | DDR_DQ27
L25 | DDR_DQ28
N25 | DDR_DQ29
N26 | DDR_DQ30
P25 | DDR_DQ31
AB25 | DDR_DQM0
U26 | DDR_DQM1
G27 | DDR_DQM2
M25 | DDR_DQM3
AA26 | DDR_DQS0N
AA25 | DDR_DQS0P
R25 | DDR_DQS1N
T25 | DDR_DQS1P
F26 | DDR_DQS2N
F27 | DDR_DQS2P
L27 | DDR_DQS3N
L26 | DDR_DQS3P
E21 | DDR_RESETN
G21 | DDR_VREF
K22 | DDR_ZQ
C8 | DSI_CKN
C7 | DSI_CKP
C9 | DSI_D0N
B9 | DSI_D0P
A10 | DSI_D1N
B10 | DSI_D1P
A7 | DSI_D2N
B7 | DSI_D2P
B6 | DSI_D3N
A6 | DSI_D3P
D6 | DSI_REXT
AA5 | JTCK_SWCLK
AE3 | JTDI
AC2 | JTDO_TRACESWO
AE2 | JTMS_SWDIO
G3 | LVDS1_D0N
G2 | LVDS1_D0P
H4 | LVDS1_D1N
H3 | LVDS1_D1P
J2 | LVDS1_D2N
J1 | LVDS1_D2P
L3 | LVDS1_D3N
L2 | LVDS1_D3P
K2 | LVDS1_D4N
K1 | LVDS1_D4P
B2 | LVDS2_D0N
B1 | LVDS2_D0P
C3 | LVDS2_D1N
C2 | LVDS2_D1P
D3 | LVDS2_D2N
E3 | LVDS2_D2P
E2 | LVDS2_D3N
E1 | LVDS2_D3P
F2 | LVDS2_D4N
F1 | LVDS2_D4P
AF3 | NJTRST
AE1 | NRST
W3 | NRSTC1MS
AA2 | OSC32_IN
AA1 | OSC32_OUT
AG2 | OSC_IN
AF2 | OSC_OUT
AF5 | PA0
AC19 | PA1
AF17 | PA2
AD18 | PA3
AG17 | PA4
AE17 | PA5
AF18 | PA6
AE18 | PA7
AA17 | PA8
AF15 | PA9
AE15 | PA10
AD12 | PA11
AC13 | PA12
AD14 | PA13
AB12 | PA14
AE13 | PA15
B13 | PB0
C12 | PB1
A14 | PB2
B14 | PB3
B15 | PB4
C14 | PB5
C13 | PB6
C11 | PB7
D8 | PB8
F10 | PB9
B11 | PB10
A11 | PB11
C26 | PB12
A26 | PB13
C27 | PB14
AE6 | PB15
AB14 | PC0
AG14 | PC1
AE12 | PC2
AA9 | PC3
AC9 | PC4
AD10 | PC5
AB10 | PC6
AF9 | PC7
AG9 | PC8
AE9 | PC9
AG10 | PC10
AD8 | PC11
AE7 | PC12
W7 | PC13
AE26 | PCIE_CLKINN
AE25 | PCIE_CLKINP
AG26 | PCIE_CLKOUTN
AF26 | PCIE_CLKOUTP
B17 | PD0
A19 | PD1
D12 | PD2
G13 | PD3
C18 | PD4
B18 | PD5
A18 | PD6
D20 | PD7
C16 | PD8
C15 | PD9
C17 | PD10
A15 | PD11
B26 | PD12
D25 | PD13
E19 | PD14
E15 | PD15
W2 | PDR_ON
B19 | PE0
C19 | PE1
C20 | PE2
C21 | PE3
B21 | PE4
C22 | PE5
A22 | PE6
B22 | PE7
C23 | PE8
A23 | PE9
D22 | PE10
B23 | PE11
C25 | PE12
C24 | PE13
B25 | PE14
D24 | PE15
AA15 | PF0
AE11 | PF1
AC15 | PF2
AF11 | PF3
AF10 | PF4
AA11 | PF5
AC7 | PF6
AB8 | PF7
AE10 | PF8
AE8 | PF9
AE5 | PF10
AE4 | PF11
P4 | PF12
P2 | PF13
P3 | PF14
R2 | PF15
AF7 | PG0
AD4 | PG1
AG5 | PG2
AA7 | PG3
AD6 | PG4
R3 | PG5
T3 | PG6
U2 | PG7
L5 | PG8
M3 | PG9
M4 | PG10
N2 | PG11
N3 | PG12
P1 | PG13
N1 | PG14
K6 | PG15
AC17 | PH2
AE19 | PH3
AB16 | PH4
AG18 | PH5
AF19 | PH6
AE16 | PH7
AD16 | PH8
AA13 | PH9
AF14 | PH10
AE14 | PH11
AF13 | PH12
AG13 | PH13
L7 | PI0
M6 | PI1
N5 | PI2
N7 | PI3
P6 | PI4
K4 | PI5
J3 | PI6
J5 | PI7
U5 | PI8
U1 | PI9
D16 | PI10
B27 | PI11
AB4 | PWR_CPUON
AF1 | PWR_LP
AD3 | PWR_ON
T4 | PZ0
U7 | PZ1
W5 | PZ2
Y6 | PZ3
V3 | PZ4
R5 | PZ5
V4 | PZ6
V2 | PZ7
V1 | PZ8
U3 | PZ9
AB18 | UCPD1_CC1
AA19 | UCPD1_CC2
AG22 | USB3DR_DM
AF22 | USB3DR_DP
AF23 | USB3DR_TXRTUNE
AD20 | USB3DR_VBUS
AG21 | USBH_HS_DM
AF21 | USBH_HS_DP
AE20 | USBH_HS_TXRTUNE
R7 | V08CAP
T6 | VBAT
AE22 | VDD33UCPD
AE21 | VDD33USB
1L1 | VDD
AB6 | VDDA18ADC
AB3 | VDDA18AON
AE23 | VDDA18COMBOPHY
G7 | VDDA18CSI
F20 | VDDA18DDR
G9 | VDDA18DSI
G5 | VDDA18LVDS
G19 | VDDA18PLL1
H6 | VDDA18PLL2
1E1 | VDDA18PLL3
AD22 | VDDA18USB
AB20 | VDDCOMBOPHY
AB22 | VDDCOMBOPHYTX
1C1 | VDDCORE
1C7 | VDDCPU
E5 | VDDCSI
F8 | VDDDSI
1G7 | VDDGPU
D14 | VDDIO1
D18 | VDDIO2
D10 | VDDIO3
E9 | VDDIO4
F4 | VDDLVDS
AC21 | VDDPCIECLK
1C11 | VDDQDDR
AF6 | VREFN
AG6 | VREFP
1A1 | VSS
AC5 | VSSA
AC3 | VSSAON
|[Merged Pins]  1L1
|1L3  |  VDD
|1L5  |  VDD
|1M2  |  VDD
|1M4  |  VDD
|[Merged Pins]  1C1
|1C3  |  VDDCORE
|1C5  |  VDDCORE
|1D2  |  VDDCORE
|1D4  |  VDDCORE
|1E3  |  VDDCORE
|1E5  |  VDDCORE
|1F2  |  VDDCORE
|1F4  |  VDDCORE
|[Merged Pins]  1C7
|1C9  |  VDDCPU
|1D6  |  VDDCPU
|1D8  |  VDDCPU
|1D10  |  VDDCPU
|F18  |  VDDCPU
|G15  |  VDDCPU
|G17  |  VDDCPU
|[Merged Pins]  1G7
|1G9  |  VDDGPU
|1H6  |  VDDGPU
|1H8  |  VDDGPU
|1H10  |  VDDGPU
|1L7  |  VDDGPU
|1L9  |  VDDGPU
|1M6  |  VDDGPU
|1M8  |  VDDGPU
|1M10  |  VDDGPU
|[Merged Pins]  D14
|E13  |  VDDIO1
|[Merged Pins]  D18
|E17  |  VDDIO2
|[Merged Pins]  D10
|E11  |  VDDIO3
|[Merged Pins]  E9
|G11  |  VDDIO4
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[Model Data]
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[End Model Data]
[End Package Model]
|End [Component]
| Models and submodels in the file (84): synopsys_usb3_tx (Output), synopsys_usb3_rx (Input), USB2_HSRX (Input), USB2_HSTX_00_0_01_0011_11 (Output), USB2_HSTX_00_0_10_0101_11 (Output), USB2_HSTX_00_0_11_0111_11 (Output), USB2_HSTX_00_1_01_0011_11 (Output), USB2_HSTX_00_1_10_0101_11 (Output), USB2_HSTX_00_1_11_0111_11 (Output), USB2_HSTX_01_0_01_0011_11 (Output), USB2_HSTX_01_0_10_0101_11 (Output), USB2_HSTX_01_0_11_0111_11 (Output), USB2_HSTX_01_1_01_0011_11 (Output), USB2_HSTX_01_1_10_0101_11 (Output), USB2_HSTX_01_1_11_0111_11 (Output), USB2_HSTX_10_0_01_0011_11 (Output), USB2_HSTX_10_0_10_0101_11 (Output), USB2_HSTX_10_0_11_0111_11 (Output), USB2_HSTX_10_1_01_0011_11 (Output), USB2_HSTX_10_1_10_0101_11 (Output), USB2_HSTX_10_1_11_0111_11 (Output), DPHY_TX_2P5G (Output), DPHY_TX_1P5G (Output), DPHY_RX_1P5G_L1 (Input), DPHY_RX_2P5G_L1 (Input), io8_tt_fs_3v3 (I/O), io8_tt_hs_3v3 (I/O), io8_tt_hslv_fs_1v8 (I/O), io8_tt_hslv_hs_1v8 (I/O), io8_tt_hslv_ls_1v8 (I/O), io8_tt_hslv_ms_1v8 (I/O), io8_tt_i3c_3v3 (I/O_open_drain), io8_tt_ls_3v3 (I/O), io8_tt_ms_3v3 (I/O), isudq_tt_1v8 (Input), isudq_tt_3v3 (Input), mal4drv20_d3_20 (I/O), mal4drv20_d3_24 (I/O), mal4drv20_d3_30 (I/O), mal4drv20_d3_40 (I/O), mal4drv20_d3_60 (I/O), mal4drv20_d4_20 (I/O), mal4drv20_d4_24 (I/O), mal4drv20_d4_30 (I/O), mal4drv20_d4_40 (I/O), mal4drv20_d4_60 (I/O), mal4drv20_dl4_20 (I/O), mal4drv20_dl4_24 (I/O), mal4drv20_dl4_30 (I/O), mal4drv20_dl4_40 (I/O), mal4drv20_dl4_60 (I/O), mal4drv27_d3_28 (I/O), mal4drv27_d3_34 (I/O), mal4drv27_d3_40 (I/O), mal4drv27_d3_53 (I/O), mal4drv27_d3_odt120 (Input), mal4drv27_d3_odt60 (Input), mal4drv27_dl4_28 (I/O), mal4drv27_dl4_34 (I/O), mal4drv27_dl4_40 (I/O), mal4drv27_dl4_53 (I/O), mal4drv27_dl4_odt48 (Input), mal4drv27_dl4_odt60 (Input), mal4drv27_d4_28 (I/O), mal4drv27_d4_34 (I/O), mal4drv27_d4_40 (I/O), mal4drv27_d4_53 (I/O), mal4drv27_d4_odt120 (Input), mal4drv27_d4_odt240 (Input), mal4drv27_d4_odt48 (Input), mal4drv27_d4_odt60 (Input), mal4drv27_d4_odt80 (Input), mal4drv20_d3l_120 (I/O), mal4drv20_d3l_40 (I/O), mal4drv20_d3l_60 (I/O), mal4drv27_d3l_120 (I/O), mal4drv27_d3l_240 (I/O), mal4drv27_d3l_40 (I/O), mal4drv27_d3l_48 (I/O), mal4drv27_d3l_60 (I/O)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
